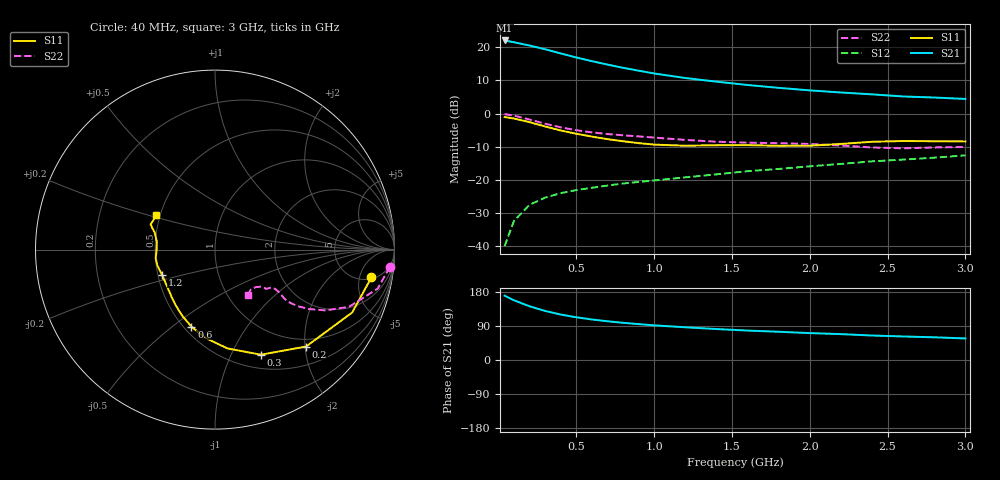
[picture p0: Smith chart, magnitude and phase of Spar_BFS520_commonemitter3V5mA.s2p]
! Filename:  BFS520B.S2P  Version:  4.0
! NXP part #: BFS520  Date: Jun 1994
! Bias condition: Vce=3V, Ic=5mA
#  MHz  S  MA  R  50
! Freq  S11  S21  S12  S22  !GUM [dB]
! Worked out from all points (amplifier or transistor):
!   21 points, 40 MHz to 3 GHz, reference 50 ohm
!   highest |S21| = 22.0 dB at 40 MHz (marker M1)
!   |S21| within 3 dB of that: start of sweep to 327.9 MHz
!   unconditionally stable (mu >= 1): 1.028 GHz to end of sweep
!   at 300 MHz: K = 0.45, MSG = 22.4 dB, |S12| = -25.4 dB
!   at 1 GHz: K = 0.99, MSG = 16.1 dB, |S12| = -20.2 dB
!   at 3 GHz: K = 1.09, MAG = 6.7 dB, |S12| = -12.6 dB
!   lowest NFmin = 0.90 dB at 500 MHz
!   S11 on the Smith chart (normalised r, x): 40 MHz: 5.33, -7.64; 200 MHz: 0.84, -2.02; 300 MHz: 0.66, -1.31; 600 MHz: 0.55, -0.59; 1.2 GHz: 0.53, -0.16; 3 GHz: 0.48, +0.21
40  0.885 -10.1  12.64 169.8  0.01 83.8  0.979 -5.7
100  0.841 -24.6  11.87 157.6  0.024 74.5  0.932 -13.5
200  0.741 -46.8  10.6 141.8  0.042 64.1  0.812 -23.1
300  0.639 -66.4  9.319 129.5  0.054 58.5  0.703 -28.8
400  0.555 -82.8  8.055 119.9  0.063 55.7  0.62 -32.3
500  0.496 -95.9  7.005 112.8  0.07 54.6  0.56 -34.3
600  0.449 -107.0  6.167 107.0  0.076 54.7  0.52 -35.2
700  0.411 -116.4  5.475 102.2  0.082 55.4  0.491 -35.5
800  0.382 -124.5  4.898 98.2  0.088 56.4  0.47 -35.1
900  0.358 -132.4  4.426 94.7  0.093 57.5  0.452 -34.5
1000  0.34 -140.3  4.022 91.5  0.098 58.5  0.434 -33.8
1200  0.327 -154.7  3.431 86.3  0.109 60.6  0.4 -33.1
1400  0.333 -164.8  3.025 81.7  0.121 63.0  0.376 -34.2
1600  0.334 -171.7  2.694 77.7  0.135 64.2  0.364 -36.6
1800  0.326 -178.5  2.438 74.5  0.146 66.1  0.357 -37.6
2000  0.327 172.3  2.235 71.0  0.16 67.2  0.348 -37.8
2200  0.348 164.5  2.076 68.3  0.174 68.6  0.329 -38.9
2400  0.375 160.2  1.946 64.6  0.19 69.1  0.308 -42.8
2600  0.385 158.6  1.808 62.1  0.202 69.3  0.299 -48.5
2800  0.382 155.8  1.743 59.9  0.216 70.3  0.308 -52.6
3000  0.379 149.9  1.66 56.9  0.234 70.5  0.313 -54.2
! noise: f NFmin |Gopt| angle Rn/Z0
500  0.9  0.325  31  0.2
900  1.1  0.266  54  0.21
2000  1.94  0.245  174  0.17
